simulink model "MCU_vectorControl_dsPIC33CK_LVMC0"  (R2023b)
settings: Solver=FixedStepDiscrete  StartTime=0.0  StopTime=10.0  FixedStep=5e-5  RelTol=1e-3  EnableMultiTasking=on
undefined symbols (not defined in the file or in its folder): A0, A4, ADC, address, also, AN0, AN1, as, B0, B2, below, Bias1, Bias2, bit, bits, BOR, C12, C13, C14, C7, C8, cause, Code, Communicate, control, counter, Custom, D11, D12, D13, D14, D2, D5, D6, D7, D9, dead, default, deviced, diff, disasserted, DiscIntNeverNeededParam, ECIO, ensure, events, faster, HS3, I, I2C, I2C1, I2C2, I2C3, illegalInstruction, Interval, inverter, is, IsSigned1, IsSigned2, kHz, Lowest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
libraries: simulink x55, MCHP_Blockset x25
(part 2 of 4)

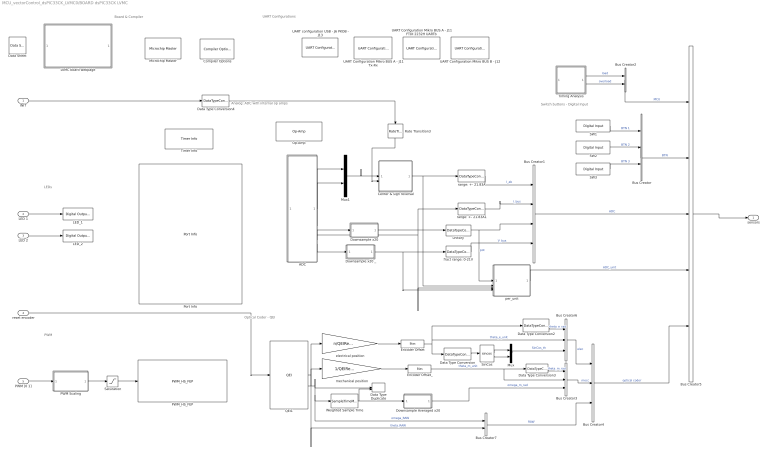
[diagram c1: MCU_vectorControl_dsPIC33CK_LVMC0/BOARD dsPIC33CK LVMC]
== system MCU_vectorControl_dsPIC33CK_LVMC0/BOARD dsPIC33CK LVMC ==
  note: Board & Compiler
  note: Analog: ADC with internal op amps
  note: Optical Coder - QEI
  note: PWM
  note: UART Configurations
  note: LEDs
  note: Switch buttons - Digital Input
  INIT : Inport
  LED 1 : Inport  Port=2
  LED 2 : Inport  Port=3
  reset encoder : Inport  Port=4
  PWM [0 1] : Inport  Port=5  Unit=1
  ADC : Subsystem
  Bus Creator{,3..4,6} (4 alike) : BusCreator  Inputs=3
  Bus Creator1 : BusCreator  Inputs=4
  Bus Creator2 : BusCreator  Inputs=2
  Bus Creator5 : BusCreator  Inputs=5
  Bus Creator7 : BusCreator  Inputs=2
  Center & sign reversal : Subsystem
  Compiler Options : MCHP_Blockset/System Configuration/Compiler Options  Priority=1  LATEST_CMPLR=on  COMP_LIST_TXT=XC16 - v2.10  DFP_LIST_TXT=from compiler  CMSIS_DSP_TXT=Dynamic Options  USE_64BIT_DOUBLE=off  MCHP_MULTITHREAD_COMPILATION=on  UseCustom_LinkerScript=off  MCHP_MASTERLINK=MCU_vectorControl_dsPIC33CK_LVMC0/BOARD dsPIC33CK LVMC/Microchip Master  OPTIMIZATION_LEVEL=2  MPLAB_LINKLIB=relaxed floating-point math  MPLAB_LINKLIB1=default  CodeReplacement_TXT=Microchip Code Replacement Library for dsPIC  OPTIMIZATION_FLTO=on  OPTIMIZATION_REORDER=off  OPTIMIZATION_ASM_REORDER=off  UNROLL_LOOPS=off  PROCEDURAL_ABSTRACTION=off  GC_SECTIONS=None  MCODE=is more than 32768  MCONST=in code memory  MDATA=Can use all available memory  MSCALAR=Use only memory below address 8192 (faster)  MLARGEARRAY=off  MAGGREGATE=on  HEAP_SIZE=0  OMF=elf  DEBUG_INFO=on  MCHP_STACK_USAGE=off  GCC_STACK_USAGE=off  ProduceHexOutput=on  AssemblyListing=off  SaveTemps=off  NO_EDS_WARN=on  PRINT_STATISTICS=off
  Data Sheet : MCHP_Blockset/System Info/Data Sheet  DOC_Type=datasheet  DOC_MCHP_Id=33FJ64MC802  DOC_FileLastCheckTime=[0 0 0 0 0 0]  cpy_MCHP_Id=33CK256MP508  MCHP_MASTERLINK=MCU_vectorControl_dsPIC33CK_LVMC0/BOARD dsPIC33CK LVMC/Microchip Master
  Data Type Duplicate : DataTypeDuplicate
  Data Type Conversion : DataTypeConversion
  Data Type Conversion2 : DataTypeConversion  OutDataTypeStr=fixdt(1,16,(2*pi)/2^16,0)  ConvertRealWorld=Stored Integer (SI)
  Data Type Conversion3 : DataTypeConversion  OutDataTypeStr=fixdt(1,16,(2*pi)/2^16,0)  ConvertRealWorld=Stored Integer (SI)
  Data Type Conversion4 : DataTypeConversion  OutDataTypeStr=boolean
  Downsample Averaged x20 : Subsystem  mask{DownSample=10}
      mask prompts: DownSample "DownSample Factor"
  Downsample x20 : Subsystem  mask{DownSample=20}
      mask prompts: DownSample "DownSample Factor"
  Downsample x20 _ : Subsystem  mask{DownSample=20}
      mask prompts: DownSample "DownSample Factor"
  Encoder Offset : Bias  Bias=mod(1,round((n*QEIOffset)/(2*pi)))
  Encoder Offset_ : Bias  Bias=mod(1,round(QEIOffset/(2*pi)))
  LED_1 : MCHP_Blockset/Digital IO/Digital Output Write  PORT_TXT="E   [ 0 : 15 ]"  PIN=6  INIT_VALUE=-1  PACK=off  OUTPUT_PIN_MODE=Push-Pull (default)  SIMULTANEOUS=off  ORDERING=None  SampleTime=-1  MCHP_PORT={Digital Out}{DOU}1:1:E6;  MCHP_MASTERLINK=MCU_vectorControl_dsPIC33CK_LVMC0/BOARD dsPIC33CK LVMC/Microchip Master
  LED_2 : MCHP_Blockset/Digital IO/Digital Output Write  PORT_TXT="E   [ 0 : 15 ]"  PIN=7  INIT_VALUE=-1  PACK=off  OUTPUT_PIN_MODE=Push-Pull (default)  SIMULTANEOUS=off  ORDERING=None  SampleTime=-1  MCHP_PORT={Digital Out}{DOU}1:1:E7;  MCHP_MASTERLINK=MCU_vectorControl_dsPIC33CK_LVMC0/BOARD dsPIC33CK LVMC/Microchip Master
  LVMC board webpage : Subsystem
  Microchip Master : MCHP_Blockset/System Configuration/Microchip Master  Priority=1  PICREF=33CK256MP508  TIMESTEP_REF=PWM1 Trigger 1 + ADC  BUSYFLAG=Dynamic Options  BUSYFLAG_TXT=None  VDD_range=Dynamic Options  PWRTEN=Not used  BOREN=Disable  BODENV=2.7V  BORV=Not used  FPWRT=128ms  DSBOREN=Enable ZPBOR during Deep Sleep Mode  DSLPBOR=Not used  MCLRE=Enabled  SMCLR=MCLR pin generates a normal system Reset  PMDL1WAY=Allow only one reconfiguration  RSTPRI=Device will obtain reset instruction from Primary flash  TEMP=Not used  SOSCSRC=Not used  SOSCSEL=Not used  IOL1WAY=Allow only one reconfiguration  ALTVREF=Not used  DISUVREG=Not used  DSSWEN=Not used  LPCFG=Not used  RTCBAT=Not used  VBTBOR=Not used  WUTSEL=Not used  POWERSAVE=off  FNOSC=Internal Fast RC (FRC)  FPR=ECIO w/ PLL 16x  FOSFPR=HS3 w/PLL 16x  FOS=Primary Oscillator  FRANGE=High Range  OSCILLATOR_SELECT=Internal Fast RC (FRC)  OSCILLATOR_SELECT_spd=Internal Fast RC (FRC)  QUARTZ=8e6  QUARTZ_spd=8e6  POSCGAIN=2x gain setting  POSCBOOST=Boost the kick start of the oscillator  SOSCGAIN=2x gain setting  SOSCBOOST=Boost the kick start of the oscillator  ACTIV_PLL=on  ACTIV_PLL_spd=on  MIPS_DESIRED=100e6  MIPS_DESIRED_spd=100e6  CPUDIV=Divide by 1  FPLLMUL=Not used  FPLLIDIV=8x Divider  POSCFREQ=Not used  POSCMD=Primary Oscillator Disabled  POSCMOD=Primary Oscillator Disabled  MIPS=100 * 1e6  ACLKCON=Optimized for PWM resolution & ADC conversion speed  ACLKCON_spd=Optimized for PWM resolution & ADC conversion speed  FPLLODIV=32x Divider  PLLKEN=PLL lock signal will be used to disable PLL clock output if lock is lost  FCKSM=Clock switching is enabled;Fail-safe Clock Monitor is disabled  FCKSMEN=Sw Disabled; Mon Disabled  IESO=Start up with FRC; then switch  DSWDTPS=1:2^36  FWDTEN=WDT controlled via SW; use WDTCON.ON bit  FWDTWINSZ=Window size is 25%  FWPSA=1:512  FWPSA0=1:128  FWPSB=1:16  WDT=Disable  WDTPOST=1:32768  WDTPRE=1:128  WDTPS=1:32768  WINDIS=Watchdog Timer operates in Non-Window mode  WWDTEN=Non-Window mode  DSWDTEN=Enable DSWDT during Deep Sleep Mode  DSWDTOSC=Select LPRC as DSWDT Reference clock  FWDT_RCLKSEL=WDT Run Mode uses BFRC:256  FWDT_RWDTPS=1:2147483648  FWDT_SWDTMPS=1:2147483648  FWDT_WDTEN=WDT is controlled by software; use WDTCON.ON bit  FWDT_WDTRSTEN=WDT event generates a reset  FWDT_WDTWIN=WDT Window is 25% of WDT period  FWDT_WINEN=Not used  FPBDIV=Not used  FSOSCEN=Disable Secondary Oscillator  LPRCSEL=Not used  OSCIOFCN=Not used  OSCIOFNC=general purpose digital I/O pin  LVRCFG=Not used  PLL_96MHZ=Not used  PLL96MHZ=Not used  PLLDIV=Not used  WDTCLK=Not used  WDTCMX=Not used  WDTWIN=WDT Window is 25% of WDT period  XTCFG=24-32 MHz crystals  XTBST=Boost the kick-start  APL=Aux Flash Code protect is disabled  APLK=Aux Flash Write Protection or Code Protection is Enabled  AWRP=Auxiliary program memory is not write-protected  BSS=No Protection (other than BWRP)  BWP=Not used  BWRP=Boot Segment may be written  CP=Protection Disabled  EBS=No Boot EEPROM  ESS=No Segment Data EEPROM  GCP=General Segment Code protect is Disabled  GSS=No Protection (other than GWRP)  GSS0=Not used  GSSK=General Segment Write Protection or Code Protection is Enabled  GWRP=General Segment may be written  PWP=Not used  RBS=No Boot RAM  RSS=No Secure RAM  SSS=No Secure Segment  SWRP=Secure segment may be written  WPCFG=Not used  WPDIS=Not used  WPEND=Not used  WPFP=Not used  ICESEL=Communicate on PGEC1/PGED1  ICS=Communicate on PGC3 and PGD3  JTAGEN=Disable  FICD_JTAGEN=Disable  COE=Not used  RES=Not used  DEBUG=Debugger is disabled  BACKBUG=Not used  BKBUG=Not used  ALTI2C=I2C mapped to SDA1/SCL1 pins  ALTI2C1=I2C1 mapped to SDA1/SCL1 pins  ALTI2C2=I2C2 mapped to SDA2/SCL2 pins  ALTI2C3=I2C3 mapped to SDA3/SCL3 pins  FDEVOPT1_ALTI2C1=Not used  FDEVOPT1_ALTI2C2=Not used  FDEVOPT1_SPI2MAPDIS=Not used  FDEVOPT_ALTI2C1=Primary I2C1 pins are used  FDEVOPT_ALTI2C2=Primary I2C2 pins are used  FDEVOPT_ALTI2C3=Primary I2C3 pins are used  FDEVOPT_SPI2PIN=SPI2 pins are selected by peripheral pin selection feature  ALTQIO=QEA1; QEB1; INDX1 are selected as inputs to QEI1  ALTSS1=SS1A is selected as the I/O pin for SPI1  CMPPOL0=Hysteresis is applied to falling edge  CMPPOL1=Hysteresis is applied to falling edge  FCANIO=Not used  FETHIO=Default Ethernet I/O  FMIIEN=MII Enabled  FSRSSEL=Not used  FUSBIDIO=Controlled by the USB Module  FVBUSONIO=Not used  HPOL=PWM module high side output pins have active-high output polarity  HYST0=45 mV Hysteresis  HYST1=45 mV Hysteresis  I2C1SEL=Not used  LPOL=PWM module low side output pins have active-high output polarity  PWMPIN=PWM module pins controlled by PORT register at device Reset  RTCOSC=Not used  UPLLEN=USB PLL Disabled  UPLLIDIV=Not used  ATMOD8=Not used  ALTPMP=Not used  I2C2SEL=Not used  ALTADREF=Not used  ALTCVREF=Not used  PWMLOCK=PWM registers may be written without key sequence  INT_PRIORITY_DMA=0  MCHP_TIMER_RESULT=[ ]  MCHP_PLLRegisters="[1    100  16387     -1     33]"  MCHPVAR=MCHP.fcy.MIPS=1e+08;MCHP.fcy.SYSCLK=1e+08;MCHP.fcy.Fplli=8000000;MCHP.fcy.Fvco=8e+08;MCHP.fcy.Fpllo=4e+08;MCHP.fcy.ADC=1e+08;MCHP.fcy.Comparator=1e+08;MCHP.fcy.I2C=1e+08;MCHP.fcy.SPI=1e+08;MCHP.fcy.UART=2e+08;MCHP.fcy.Timers=1e+08;MCHP.fcy.OC=1e+08;MCHP.fcy.IC=1e+08;MCHP.fcy.Ports=1e+08;MCHP.fcy.QEI=1e+08;MCHP.fcy.APLL=-1;MCHP.PowerSave=0;MCHP.TimeStepFactor=-20000;MCHP.TimeStep_Timer=-1;MCHP.NTIM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  MCHP_CRC=20015258  BTMODE=Device is in Single Boot (legacy) mode  RES1=Not used  PLLSS=Not used  RES2=Not used  ALTCMPI=Not used  BOREN1=Not used  ALTRB6=Not used  RETCFG=Not used  DFMCY=Not used  BSS2=No Boot Segment  BSEN=No Boot Segment  CWRP=Configuration Segment may be written  CSS=No Protection (other than CWRP)  AIVTDIS=Disabled AIVT  BSLIM=Not used  WDTEN=Disable  BTSWP=BOOTSWP instruction is disabled  DBCC=No Cross Connection between DAC outputs  CTXT1=Not Assigned  CTXT2=Not Assigned  SEQNUM=Not used  nSEQNUM=Not used  BOREN0=Enabled  DMTIVT=Not used  DMTCNT=2^31 (2147483648)  DMTEN=Dead Man Timer is Disabled and can be enabled by software  ON=Not used  USERID=Not used  RESERVED1=Not used  PGL1WAY=Allow only one reconfiguration  FPLLRNG=34-68 MHz Input  FPLLICLK=FRC is input to the System PLL  FPLLMULT=PLL Multiply by 128  UPLLFSEL=USB PLL input is 24 MHz  DMTINTV=Window/Interval value is 127/128 counter value  WDTSPGM=WDT stops during Flash programming  FDMTEN=Deadman Timer is disabled  TRCEN=Trace features in the CPU are enabled  BOOTISA=Boot code and Exception code is MIPS32  FECCCON=ECC and Dynamic ECC are disabled (ECCCON bits are writable)  EXTDDRSIZE=Not used  FSLEEP=Flash is powered down when the device is in Sleep mode  DBGPER=Allow CPU access to all permission regions  EJTAGBEN=Normal EJTAG functionality  TSEQ=Not used  CSEQ=Not used  RWDTPS=1:1048576  RCLKSEL=Always use LPRC  SWDTPS=1:1048576  DMTIVTL=Not used  DMTIVTH=Not used  DMTCNTL=Not used  DMTCNTH=Not used  DMTDIS=Dead Man Timer is Disabled and can be enabled by software  SMBEN=SMBus input threshold is enabled  SPI2PIN=SPI2 uses I/O remap (PPS) pins  CTXT3=Not Assigned  CTXT4=Not Assigned  MBXM0=Mailbox register configured for Main data read (Secondary to Main data transfer)  MBXM1=Mailbox register configured for Main data read (Secondary to Main data transfer)  MBXM2=Mailbox register configured for Main data read (Secondary to Main data transfer)  MBXM3=Mailbox register configured for Main data read (Secondary to Main data transfer)  MBXM4=Mailbox register configured for Main data read (Secondary to Main data transfer)  MBXM5=Mailbox register configured for Main data read (Secondary to Main data transfer)  MBXM6=Mailbox register configured for Main data read (Secondary to Main data transfer)  MBXM7=Mailbox register configured for Main data read (Secondary to Main data transfer)  MBXM8=Mailbox register configured for Main data read (Secondary to Main data transfer)  MBXM9=Mailbox register configured for Main data read (Secondary to Main data transfer)  MBXM10=Mailbox register configured for Main data read (Secondary to Main data transfer)  MBXM11=Mailbox register configured for Main data read (Secondary to Main data transfer)  MBXM12=Mailbox register configured for Main data read (Secondary to Main data transfer)  MBXM13=Mailbox register configured for Main data read (Secondary to Main data transfer)  MBXM14=Mailbox register configured for Main data read (Secondary to Main data transfer)  MBXM15=Mailbox register configured for Main data read (Secondary to Main data transfer)  MBXHSA=MSIxMBXD15 assigned to mailbox handshake protocol block A  MBXHSB=MSIxMBXD15 assigned to mailbox handshake protocol block B  MBXHSC=MSIxMBXD15 assigned to mailbox handshake protocol block C  MBXHSD=MSIxMBXD15 assigned to mailbox handshake protocol block D  MBXHSE=MSIxMBXD15 assigned to mailbox handshake protocol block E  MBXHSF=MSIxMBXD15 assigned to mailbox handshake protocol block F  MBXHSG=MSIxMBXD15 assigned to mailbox handshake protocol block G  MBXHSH=MSIxMBXD15 assigned to mailbox handshake protocol block H  HSAEN=Mailbox data flow control handshake protocol block disabled  HSBEN=Mailbox data flow control handshake protocol block disabled  HSCEN=Mailbox data flow control handshake protocol block disabled  HSDEN=Mailbox data flow control handshake protocol block disabled  HSEEN=Mailbox data flow control handshake protocol block disabled  HSFEN=Mailbox data flow control handshake protocol block disabled  HSGEN=Mailbox data flow control handshake protocol block disabled  HSHEN=Mailbox data flow control handshake protocol block disabled  CPRA0=Main core owns pin  CPRA1=Main core owns pin  CPRA2=Main core owns pin  CPRA3=Main core owns pin  CPRA4=Main core owns pin  CPRB0=Main core owns pin  CPRB1=Main core owns pin  CPRB2=Main core owns pin  CPRB3=Main core owns pin  CPRB4=Main core owns pin  CPRB5=Main core owns pin  CPRB6=Main core owns pin  CPRB7=Main core owns pin  CPRB8=Main core owns pin  CPRB9=Main core owns pin  CPRB10=Main core owns pin  CPRB11=Main core owns pin  CPRB12=Main core owns pin  CPRB13=Main core owns pin  CPRB14=Main core owns pin  CPRB15=Main core owns pin  CPRC0=Main core owns pin  CPRC1=Main core owns pin  CPRC2=Main core owns pin  CPRC3=Main core owns pin  CPRC4=Main core owns pin  CPRC5=Main core owns pin  CPRC6=Main core owns pin  CPRC7=Main core owns pin  CPRC8=Main core owns pin  CPRC9=Main core owns pin  CPRC10=Main core owns pin  CPRC11=Main core owns pin  CPRC12=Main core owns pin  CPRC13=Main core owns pin  CPRC14=Main core owns pin  CPRC15=Main core owns pin  CPRD0=Main core owns pin  CPRD1=Main core owns pin  CPRD2=Main core owns pin  CPRD3=Main core owns pin  CPRD4=Main core owns pin  CPRD5=Main core owns pin  CPRD6=Main core owns pin  CPRD7=Main core owns pin  CPRD8=Main core owns pin  CPRD9=Main core owns pin  CPRD10=Main core owns pin  CPRD11=Main core owns pin  CPRD12=Main core owns pin  CPRD13=Main core owns pin  CPRD14=Main core owns pin  CPRD15=Main core owns pin  CPRE0=Main core owns pin  CPRE1=Main core owns pin  CPRE2=Main core owns pin  CPRE3=Main core owns pin  CPRE4=Main core owns pin  CPRE5=Main core owns pin  CPRE6=Main core owns pin  CPRE7=Main core owns pin  CPRE8=Main core owns pin  CPRE9=Main core owns pin  CPRE10=Main core owns pin  CPRE11=Main core owns pin  CPRE12=Main core owns pin  CPRE13=Main core owns pin  CPRE14=Main core owns pin  CPRE15=Main core owns pin  S1FNOSC=Internal Fast RC (FRC) Oscillator with postscaler  S1IESO=Start up with FRC; then switch  S1OSCIOFNC=OSC2 is clock output  S1FCKSM=Both Clock switching and Fail-safe Clock Monitor are disabled  S1PLLKEN=S1PLLKEN_ON  S1RWDTPS=1:1048576  S1RCLKSEL=Always use LPRC  S1WINDIS=Watchdog Timer operates in Non-Window mode  S1WDTWIN=WDT Window is 25% of WDT period  S1SWDTPS=1:1048576  S1FWDTEN=use WDTCON.ON bit  S1ICS=Communicate on PGC3 and PGD3  S1DEBUG=Not used  S1ISOLAT=The Secondary can operate (in debug mode) even if the SLVEN bit in the MSI is zero  S1NOBTSWP=BOOTSWP instruction is disabled  S1ALTI2C1=I2C1 mapped to SDA1/SCL1 pins  S1SPI1PIN=Secondary SPI1 uses I/O remap (PPS) pins  S1SSRE=Secondary generated resets will reset the Secondary Enable Bit in the MSI module  S1MSRE=The Main software oriented RESET events (RESET Op-Code; Watchdog timeout; TRAP reset; illegalInstruction) will also cause the Secondary subsystem to reset  S1CTXT1=Not Assigned  S1CTXT2=Not Assigned  S1CTXT3=Not Assigned  S1CTXT4=Not Assigned  BORLVL=BOR trip point is 2.96 V  BSSO=Normal startup operation after reset; execute instruction at 0x000000  MCA=Flash read accesses are 2 cycle to support maximum processor frequency of operation  MAXTEMP=20 ns flash access  CFGAN14=Device pin is input to AN14  CFGAN15=Device pin is input to AN15  S1IOL1WAY=Allow only one reconfiguration  S1BSSO=Normal startup operation after reset; execute instruction at 0x000000  S1BACKBUG=Not used  BISTDIS=mBIST on reset feature disabled  NOBTSWP=BOOTSWP instruction is disabled  S1BISTDIS=Secondary BIST on reset feature disabled  S1DMTIVTL=Not used  S1DMTIVTH=Not used  S1DMTCNTL=Not used  S1DMTCNTH=Not used  S1DMTDIS=Secondary Dead Man Timer is Disabled and can be enabled by software  BSEQ=Not used  IBSEQ=Not used  SMB3EN=SMBus 3.0 input levels  FUSBIDIO2=USBID pin is controlled by the USB2 module  FVBUSIO2=VBUSON pin is controlled by the USB2 module  FUSBIDIO1=USBID pin is controlled by the USB1 module  FVBUSIO1=VBUSON pin is controlled by the USB1 module  VBATBOREN=Enable ZPBOR during VBAT Mode  FDSEN=Enable DSEN bit in DSCON  BORSEL=BOR trip voltage 2.1v (Non-OPAMP deviced operation)  POSCFGAIN=Gain is G3  POSCAGCDLY=Settling time = 25ms x AGCRNG  POSCAGCRNG=Range 1x  POSCAGC=Automatic Gain Control for Oscillator  FDBGWP=Not used
  Mux : Mux  Inputs=2
  Mux1 : Mux  Inputs=2
  Op-Amp : MCHP_Blockset/Analog IO/Op-Amp  Priority=-2000  OpAmp1=Enabled with positive and negative inputs  OpAmp2=Enabled with positive and negative inputs  OpAmp3=Enabled with positive and negative inputs  S_INPUT=[-1]  S_INPUT_Size=[3]  S_OUTPUT=[]  S_OUTPUT_Size=[]  S_ListCustomDatatype=S.S_ListCustomDatatype={};  MCHP_USER_INTERRUPTS=0  MCHP_PORT={OA1 Output}{OA1out}14:2:A0;{OA1 IN+}{OA1in+}14:2:A2;{OA1 IN-}{OA1in-}14:2:A1;{OA2 Output}{OA2out}14:2:B2;{OA2 IN+}{OA2in+}14:2:B4;{OA2 IN-}{OA2in-}14:2:B3;{OA3 Output}{OA3out}14:2:A4;{OA3 IN+}{OA3in+}14:2:C2;{OA3 IN-}{OA3in-}14:2:C1;  MCHP_MASTERLINK=MCU_vectorControl_dsPIC33CK_LVMC0/BOARD dsPIC33CK LVMC/Microchip Master  MCHP_CRC=1127818
  PWM Scaling : Subsystem
  PWM_HS_FEP : MCHP_Blockset/PWM IO/PWM_HS_FEP  Priority=-2000  PWMx_MODSEL=Center Aligned  PWMx_CLKSEL=no scaling  PWM_ClockResolution_DIVSEL_TXT=auto  PWM_ClockResolution_FSCL_TXT=auto - best resolution  PWM_ClockResolution_NoScaling_TXT="Resol: 0.005(us)  -  MaxPer: 0.000328(s)"  MaxPeriod_s=50e-6  InitPeriode_s=50e-6  InitDutyCycleP_s=25e-6  InitDutyCycleS_s=10e-6  InitPhase_s=-1  evalin_ws=PWM1max=MCHP_Fun.Hex2num('40B3880000000000');PWM2max=MCHP_Fun.Hex2num('40B3880000000000');PWM4max=MCHP_Fun.Hex2num('40B3880000000000');  SampleTime=-1  S_INPUT=[-1]  S_INPUT_Size=[3]  S_OUTPUT=[]  S_OUTPUT_Size=[]  S_ListCustomDatatype=S.S_ListCustomDatatype={};  MCHP_USER_INTERRUPTS=0  MCHP_PORT={PWMH1 }{PWMH1}32:4:B14;{PWMH2 }{PWMH2}32:4:B12;{PWMH4 }{PWMH4}32:4:D1;{PWML1}{PWML1}32:4:B15;{PWML2}{PWML2}32:4:B13;{PWML4}{PWML4}32:4:D0;  MCHP_MASTERLINK=MCU_vectorControl_dsPIC33CK_LVMC0/BOARD dsPIC33CK LVMC/Microchip Master  MCHP_CRC=5297627  PWMx_PMOD=Complementary  PWM1_HL=PWMxH & PWMxL output enabled  PWM1_swap=off  PWM1H_pol=off  PWM1L_pol=off  PWM2_HL=PWMxH & PWMxL output enabled  PWM2_swap=off  PWM2H_pol=off  PWM2L_pol=off  PWM3_HL=not used  PWM3_swap=off  PWM3H_pol=off  PWM3L_pol=off  PWM4_HL=PWMxH & PWMxL output enabled  PWM4_swap=off  PWM4H_pol=off  PWM4L_pol=off  PWM5_HL=not used  PWM5_swap=off  PWM5H_pol=off  PWM5L_pol=off  PWM6_HL=not used  PWM6_swap=off  PWM6H_pol=off  PWM6L_pol=off  PWM7_HL=not used  PWM7_swap=off  PWM7H_pol=off  PWM7L_pol=off  PWM8_HL=not used  PWM8_swap=off  PWM8H_pol=off  PWM8L_pol=off  PWM9_HL=not used  PWM9_swap=off  PWM9H_pol=off  PWM9L_pol=off  PWM10_HL=not used  PWM10_swap=off  PWM10H_pol=off  PWM10L_pol=off  PWM11_HL=not used  PWM11_swap=off  PWM11H_pol=off  PWM11L_pol=off  PWM12_HL=not used  PWM12_swap=off  PWM12H_pol=off  PWM12L_pol=off  PWM1_ShowTrig=on  PWM1_Init_PGxTRIGABC_s=[0 -1 -1 ]  PWM1_ADTRxEN1=ADC Trigger 1  PWM1_ADTRxEN2=none  PWM1_ADTRxEN3=none  PWM2_ShowTrig=off  PWM2_Init_PGxTRIGABC_s=[-1 -1 -1]  PWM2_ADTRxEN1=none  PWM2_ADTRxEN2=none  PWM2_ADTRxEN3=none  PWM3_ShowTrig=off  PWM3_Init_PGxTRIGABC_s=[-1 -1 -1]  PWM3_ADTRxEN1=none  PWM3_ADTRxEN2=none  PWM3_ADTRxEN3=none  PWM4_ShowTrig=off  PWM4_Init_PGxTRIGABC_s=[-1 -1 -1]  PWM4_ADTRxEN1=none  PWM4_ADTRxEN2=none  PWM4_ADTRxEN3=none  PWM5_ShowTrig=off  PWM5_Init_PGxTRIGABC_s=[-1 -1 -1]  PWM5_ADTRxEN1=none  PWM5_ADTRxEN2=none  PWM5_ADTRxEN3=none  PWM6_ShowTrig=off  PWM6_Init_PGxTRIGABC_s=[-1 -1 -1]  PWM6_ADTRxEN1=none  PWM6_ADTRxEN2=none  PWM6_ADTRxEN3=none  PWM7_ShowTrig=off  PWM7_Init_PGxTRIGABC_s=[-1 -1 -1]  PWM7_ADTRxEN1=none  PWM7_ADTRxEN2=none  PWM7_ADTRxEN3=none  PWM8_ShowTrig=off  PWM8_Init_PGxTRIGABC_s=[-1 -1 -1]  PWM8_ADTRxEN1=none  PWM8_ADTRxEN2=none  PWM8_ADTRxEN3=none  BlockInput_VectorScalar=Vectors (grouped by function)  BlockInput_Period=Not a block input  BlockInput_DutyCycle=a Uint raw input (PWMxmax variable represent max period)  BlockInput_PhaseShift=Not a block input  BlockInput_SEVTCMP=Not a block input  BlockInput_TRIGx=Not a block input  BlockInput_DeadTime=Not a block input  BlockOutput_FaultDisabled=off  BlockOutput_Fault=on  DTC=Positive dead time (ensure period of time with PWM_H and PWM_L disasserted)  FLTSRC1_DTCMP_TXT=<empty>  FLTSRC2_DTCMP_TXT=<empty>  FLTSRC3_DTCMP_TXT=<empty>  FLTSRC4_DTCMP_TXT=<empty>  FLTSRC5_DTCMP_TXT=<empty>  FLTSRC6_DTCMP_TXT=<empty>  FLTSRC7_DTCMP_TXT=<empty>  FLTSRC8_DTCMP_TXT=<empty>  FLTSRC9_DTCMP_TXT=<empty>  FLTSRC10_DTCMP_TXT=<empty>  FLTSRC11_DTCMP_TXT=<empty>  FLTSRC12_DTCMP_TXT=<empty>  DeadTime_s=1e-6  DeadTimeAlt_s=1e-6  DeadTimeComp_s=0  FLTMODx=Disabled  FLTSRCx_TXT=<empty>  FLTDATx=PWM H/L -> 11  CLMODx=Disabled  CLSRCx_TXT=<empty>  CLDATx=PWM H/L -> 00  FLTLEBENx=off  CLLEBENx=off  LeadEdgeBlkPer_s=5e-7  PHRx=off  PHFx=off  PLRx=off  PLFx=off
  Port Info : MCHP_Blockset/System Info/Port Info  MCHP_MASTERLINK=MCU_vectorControl_dsPIC33CK_LVMC0/BOARD dsPIC33CK LVMC/Microchip Master
  QEI1 : MCHP_Blockset/QEI/QEI  QEI_REF=1  QEI_MODE=Quadrature Encoder  QEI_x2mode=off  QEI_PulseCountDir=Down  PIN_QEA_TXT=C12 / P60 / Pin[5]  PIN_QEB_TXT=C13 / P61 / Pin[6]  SWPAB=on  QEAPOL=off  QEBPOL=off  SampleTime=50e-6  PIN_CCMP_TXT=A4 / P20 / Pin[33]  MCHP_PORT={QEI1 A}{QEIA1}5:0:P60;{QEI1 B}{QEIB1}5:0:P61;  MCHP_MASTERLINK=MCU_vectorControl_dsPIC33CK_LVMC0/BOARD dsPIC33CK LVMC/Microchip Master  INDXxCNT_Output=is not an output  POSxCNT_Output=is a 16 bits signed block output  RESET_Input=on  PIMOD_mode=position is cyclique between user defined boundaries  PIMOD_modeB=Never reset position  PIMOD_reset=on next INDEX event  PIN_INDEX_TXT=C14 / P62 / Pin[7]  IMV=QEA = 0 and QEB = 0  IMV_x2=QEA = 1  PIN_HOME_TXT=B0 / P32 / Pin[34]  QEIxLEC_GEC=[0 (QEIResolution-1)]  QEIxIC=0  PCIIRQ=off  IDXPOL=on  HOMPOL=on  VELxCNT_Output=is a 16 bits signed block output  INTxHLD_Output=is not an output  MaxPeriod=1e-3  FILTREN=on  QFDIV_popup_TXT=8333.33 kHz  FILTER_CutOffFreq=100e3  QEI_IntPri=5
  Rate Transition3 : RateTransition  Deterministic=off
  SW1 : MCHP_Blockset/Digital IO/Digital Input  PORT_TXT="E   [ 0 : 15 ]"  PIN=11  INPUT_PIN_MODE=Hi-impedance (default)  PACK=off  SIMULTANEOUS=off  ORDERING=None  SampleTime=-1  MCHP_PORT={Digital In}{DIN}2:0:E11;  MCHP_MASTERLINK=MCU_vectorControl_dsPIC33CK_LVMC0/BOARD dsPIC33CK LVMC/Microchip Master
  SW2 : MCHP_Blockset/Digital IO/Digital Input  PORT_TXT="E   [ 0 : 15 ]"  PIN=12  INPUT_PIN_MODE=Hi-impedance (default)  PACK=off  SIMULTANEOUS=off  ORDERING=None  SampleTime=-1  MCHP_PORT={Digital In}{DIN}2:0:E12;  MCHP_MASTERLINK=MCU_vectorControl_dsPIC33CK_LVMC0/BOARD dsPIC33CK LVMC/Microchip Master
  SW3 : MCHP_Blockset/Digital IO/Digital Input  PORT_TXT="E   [ 0 : 15 ]"  PIN=13  INPUT_PIN_MODE=Hi-impedance (default)  PACK=off  SIMULTANEOUS=off  ORDERING=None  SampleTime=-1  MCHP_PORT={Digital In}{DIN}2:0:E13;  MCHP_MASTERLINK=MCU_vectorControl_dsPIC33CK_LVMC0/BOARD dsPIC33CK LVMC/Microchip Master
  Saturation : Saturate  UpperLimit=PWM1max*0.97  LowerLimit=PWM1max*0.03  LinearizeAsGain=off  OutDataTypeStr=uint16
  SinCos : Trigonometry  Operator=sincos  ApproximationMethod=Lookup  AngleUnit=revolution  TableDataTypeStr=fixdt(1,16,14)
  Timer Info : MCHP_Blockset/System Info/Timer Info  MCHP_MASTERLINK=MCU_vectorControl_dsPIC33CK_LVMC0/BOARD dsPIC33CK LVMC/Microchip Master
  Timing Analysis : Subsystem
  UART Configuration Mikro BUS A - J11 FTDI 2232H UARTb : MCHP_Blockset/BUS UART/UART Configuration  UART_REF=3  BAUD_Choice_TXT="3000000         [-0.50%]"  BAUD_Choice_IR_TXT=[]  BAUD_Custom=9000000  INT_PRIORITY=0  ALT_IO=on  PIN_RX_TXT=D12 / P76 / Pin[27]  PIN_RX_INPUT_MODE=Hi-impedance (default)  PIN_TX_TXT=D11 / P75 / Pin[36]  PIN_TX_OUTPUT_MODE=Push-Pull (default)  MCHP_PORT="{UART3  Rx}{U3RX}3:0:P76;{UART3  Tx}{U3TX}3:0:P75;"  MCHP_MASTERLINK=MCU_vectorControl_dsPIC33CK_LVMC0/BOARD dsPIC33CK LVMC/Microchip Master  MCHP_COM_ExtPil=off  TX_IMPLEMENTATION=Circular Buffer  TX_IMPLEMENTATION_default=Circular Buffer  TX_INT_PRIORITY=5  TX_INT_WHEN=has one empty space  TX_INT_WHEN_default=is empty & last char is sent  TX_CIRCULAR_SIZE=1024  TX_DMA_CHANNEL=1  TX_DMA_SIZE=16  TX_TASK_PROTECTION=Delay tasks (default)  TX_INTERRUPT_PROTECTION=Do not send on conflict (default)  TX_INTERRUPT_PROTECTION_default=Do not send on conflict (default)  RX_IMPLEMENTATION=Circular Buffer  RX_IMPLEMENTATION_default=Circular Buffer  RX_INT_PRIORITY=7  RX_INT_WHEN=receive 1 character  RX_CIRCULAR_SIZE=64  RX_DMA_CHANNEL=0  RX_DMA_SIZE=0  DuplexMode=Full duplex (default)  PIN_RX_Inv=off  PIN_TX_Inv=off  PIN_RXTX_Inv=off  ParityBit=No parity (default)  StopBit=1 stop bit (default)  IRDA=off  IdleTime_choice_TXT=None  IdleTime_custom=2/50  FlowControl=None  PIN_CTS_TXT=B0 / P32 / Pin[34]  PIN_CTS_INPUT_MODE=Hi-impedance (default)  PIN_RTS_TXT=B0 / P32 / Pin[34]  PIN_RTS_OUTPUT_MODE=Push-Pull (default)  PIN_DSR_TXT=B0 / P32 / Pin[34]  PIN_DSR_INPUT_MODE=Hi-impedance (default)  PIN_DTR_TXT=B0 / P32 / Pin[34]  PIN_DTR_OUTPUT_MODE=Push-Pull (default)  InitSequence_chkbox=off  BAUD_Choice_InitSeq_TXT="110         [+73.40%]"  BAUD_Choice_IR_InitSeq_TXT=0  BAUD_Custom_InitSeq=0  InitSequence="uint8(['use VT100 terminal ! ' 13 10 27 'c'  27 '[2J' ] )"
  UART Configuration Mikro BUS A - J11 Tx-Rx : MCHP_Blockset/BUS UART/UART Configuration  UART_REF=2  BAUD_Choice_TXT="921600         [+0.01%]"  BAUD_Choice_IR_TXT=[]  BAUD_Custom=5520000  INT_PRIORITY=0  ALT_IO=on  PIN_RX_TXT=D7 / P71 / Pin[52]  PIN_RX_INPUT_MODE=Hi-impedance (default)  PIN_TX_TXT=C7 / P55 / Pin[40]  PIN_TX_OUTPUT_MODE=Push-Pull (default)  MCHP_PORT="{UART2  Rx}{U2RX}3:0:P71;{UART2  Tx}{U2TX}3:0:P55;"  MCHP_MASTERLINK=MCU_vectorControl_dsPIC33CK_LVMC0/BOARD dsPIC33CK LVMC/Microchip Master  MCHP_COM_ExtPil=off  TX_IMPLEMENTATION=DMA Circular Buffer  TX_IMPLEMENTATION_default=Circular Buffer  TX_INT_PRIORITY=5  TX_INT_WHEN=is empty & last char is sent  TX_INT_WHEN_default=is empty & last char is sent  TX_CIRCULAR_SIZE=1024  TX_DMA_CHANNEL=2  TX_DMA_SIZE=16  TX_TASK_PROTECTION=Delay tasks (default)  TX_INTERRUPT_PROTECTION=Do not send on conflict (default)  TX_INTERRUPT_PROTECTION_default=Do not send on conflict (default)  RX_IMPLEMENTATION=Circular Buffer  RX_IMPLEMENTATION_default=Circular Buffer  RX_INT_PRIORITY=7  RX_INT_WHEN=receive 1 character  RX_CIRCULAR_SIZE=64  RX_DMA_CHANNEL=0  RX_DMA_SIZE=0  DuplexMode=Full duplex (default)  PIN_RX_Inv=off  PIN_TX_Inv=off  PIN_RXTX_Inv=off  ParityBit=No parity (default)  StopBit=1 stop bit (default)  IRDA=off  IdleTime_choice_TXT=None  IdleTime_custom=2/50  FlowControl=None  PIN_CTS_TXT=B0 / P32 / Pin[34]  PIN_CTS_INPUT_MODE=Hi-impedance (default)  PIN_RTS_TXT=B0 / P32 / Pin[34]  PIN_RTS_OUTPUT_MODE=Push-Pull (default)  PIN_DSR_TXT=B0 / P32 / Pin[34]  PIN_DSR_INPUT_MODE=Hi-impedance (default)  PIN_DTR_TXT=B0 / P32 / Pin[34]  PIN_DTR_OUTPUT_MODE=Push-Pull (default)  InitSequence_chkbox=off  BAUD_Choice_InitSeq_TXT="110         [+73.40%]"  BAUD_Choice_IR_InitSeq_TXT=0  BAUD_Custom_InitSeq=0  InitSequence="uint8(['use VT100 terminal ! ' 13 10 27 'c'  27 '[2J' ] )"
  UART Configuration Mikro BUS B - J12 : MCHP_Blockset/BUS UART/UART Configuration  Commented=on  UART_REF=3  BAUD_Choice_TXT="8000000         [+0.00%]"  BAUD_Choice_IR_TXT=[]  BAUD_Custom=9000000  INT_PRIORITY=0  ALT_IO=on  PIN_RX_TXT=D5 / P69 / Pin[54]  PIN_RX_INPUT_MODE=Hi-impedance (default)  PIN_TX_TXT=D6 / P70 / Pin[53]  PIN_TX_OUTPUT_MODE=Push-Pull (default)  MCHP_PORT="{UART3  Tx}{U3TX}3:0:P70;"  MCHP_MASTERLINK=MCU_vectorControl_dsPIC33CK_LVMC0/BOARD dsPIC33CK LVMC/Microchip Master  MCHP_COM_ExtPil=off  TX_IMPLEMENTATION=Circular Buffer  TX_IMPLEMENTATION_default=Circular Buffer  TX_INT_PRIORITY=4  TX_INT_WHEN=has one empty space  TX_INT_WHEN_default=is empty & last char is sent  TX_CIRCULAR_SIZE=256  TX_DMA_CHANNEL=2  TX_DMA_SIZE=16  TX_TASK_PROTECTION=Delay tasks (default)  TX_INTERRUPT_PROTECTION=Do not send on conflict (default)  TX_INTERRUPT_PROTECTION_default=Do not send on conflict (default)  RX_IMPLEMENTATION=Do not implement Rx  RX_IMPLEMENTATION_default=Circular Buffer  RX_INT_PRIORITY=7  RX_INT_WHEN=receive 1 character  RX_CIRCULAR_SIZE=64  RX_DMA_CHANNEL=0  RX_DMA_SIZE=0  DuplexMode=Full duplex (default)  PIN_RX_Inv=off  PIN_TX_Inv=off  PIN_RXTX_Inv=off  ParityBit=No parity (default)  StopBit=1 stop bit (default)  IRDA=off  IdleTime_choice_TXT=0  IdleTime_custom=2/50  FlowControl=None  PIN_CTS_TXT=B0 / P32 / Pin[34]  PIN_CTS_INPUT_MODE=Hi-impedance (default)  PIN_RTS_TXT=B0 / P32 / Pin[34]  PIN_RTS_OUTPUT_MODE=Push-Pull (default)  PIN_DSR_TXT=Dynamic Options  PIN_DSR_INPUT_MODE=Hi-impedance (default)  PIN_DTR_TXT=Dynamic Options  PIN_DTR_OUTPUT_MODE=Push-Pull (default)  InitSequence_chkbox=off  BAUD_Choice_InitSeq_TXT="110         [+73.40%]"  BAUD_Choice_IR_InitSeq_TXT=0  BAUD_Custom_InitSeq=0  InitSequence="uint8(['use VT100 terminal ! ' 13 10 27 'c'  27 '[2J' ] )"
  UART configuration USB - J6 PKOB - J13 : MCHP_Blockset/BUS UART/UART Configuration  UART_REF=1  BAUD_Choice_TXT="460800         [+0.01%]"  BAUD_Choice_IR_TXT=[]  BAUD_Custom=115200  INT_PRIORITY=0  ALT_IO=on  PIN_RX_TXT=D14 / P78 / Pin[13]  PIN_RX_INPUT_MODE=Hi-impedance (default)  PIN_TX_TXT=D13 / P77 / Pin[14]  PIN_TX_OUTPUT_MODE=Push-Pull (default)  MCHP_PORT="{UART1  Rx}{U1RX}3:0:P78;{UART1  Tx}{U1TX}3:0:P77;"  MCHP_MASTERLINK=MCU_vectorControl_dsPIC33CK_LVMC0/BOARD dsPIC33CK LVMC/Microchip Master  MCHP_COM_ExtPil=off  TX_IMPLEMENTATION=DMA Circular Buffer  TX_IMPLEMENTATION_default=Circular Buffer  TX_INT_PRIORITY=5  TX_INT_WHEN=is empty  TX_INT_WHEN_default=is empty & last char is sent  TX_CIRCULAR_SIZE=256  TX_DMA_CHANNEL="0   (Lowest Priority)"  TX_DMA_SIZE=512  TX_TASK_PROTECTION=Delay tasks (default)  TX_INTERRUPT_PROTECTION=Do not send on conflict (default)  TX_INTERRUPT_PROTECTION_default=Do not send on conflict (default)  RX_IMPLEMENTATION=Circular Buffer  RX_IMPLEMENTATION_default=Circular Buffer  RX_INT_PRIORITY=7  RX_INT_WHEN=receive 1 character  RX_CIRCULAR_SIZE=64  RX_DMA_CHANNEL=0  RX_DMA_SIZE=0  DuplexMode=Full duplex (default)  PIN_RX_Inv=off  PIN_TX_Inv=off  PIN_RXTX_Inv=off  ParityBit=No parity (default)  StopBit=1 stop bit (default)  IRDA=off  IdleTime_choice_TXT=None  IdleTime_custom=2/50  FlowControl=None  PIN_CTS_TXT=B0 / P32 / Pin[34]  PIN_CTS_INPUT_MODE=Hi-impedance (default)  PIN_RTS_TXT=B0 / P32 / Pin[34]  PIN_RTS_OUTPUT_MODE=Push-Pull (default)  PIN_DSR_TXT=B0 / P32 / Pin[34]  PIN_DSR_INPUT_MODE=Hi-impedance (default)  PIN_DTR_TXT=B0 / P32 / Pin[34]  PIN_DTR_OUTPUT_MODE=Push-Pull (default)  InitSequence_chkbox=off  BAUD_Choice_InitSeq_TXT="115200         [+0.01%]"  BAUD_Choice_IR_InitSeq_TXT=0  BAUD_Custom_InitSeq=0  InitSequence="uint8(['use VT100 terminal ! ' 13 10 27 'c'  27 '[2J' ] )"
  Weighted Sample Time : SampleTimeMath  TsampMathOp=/  weightValue=QEIResolution / (2*pi)  OutDataTypeStr=Inherit: Inherit via back propagation
  electrical position : Gain  Gain=n/QEIResolution  OutDataTypeStr=fixdt(0,16,16)
  fract range: 0-21V : DataTypeConversion  OutDataTypeStr=fixdt(0,16,3.3/65536*21,0)  ConvertRealWorld=Stored Integer (SI)
  mechanical position : Gain  Gain=1/QEIResolution  OutDataTypeStr=fixdt(0,16,16)
  per_unit : Subsystem
  range: +- 21.83A : DataTypeConversion  OutDataTypeStr=fixdt(1,16,21.83/32768,0)  ConvertRealWorld=Stored Integer (SI)
  range: +- 21.83A1 : DataTypeConversion  OutDataTypeStr=fixdt(1,16,21.83/32768,0)  ConvertRealWorld=Stored Integer (SI)
  unitary : DataTypeConversion  OutDataTypeStr=fixdt(0,16,16)  ConvertRealWorld=Stored Integer (SI)
  sensors : Outport
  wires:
  ADC/4(pot) -> Downsample x20/1(In1)
  SW3/1 -> Bus Creator/3  "BTN 3"
  LED 2/1 -> LED_2/1
  SW2/1 -> Bus Creator/2  "BTN 2"
  QEI1/1 -> Bus Creator7/2, mechanical position/1, electrical position/1  "theta_RAW"
  Mux/1 -> Bus Creator6/3  "SinCos_th"
  mechanical position/1 -> Encoder Offset_/1
  ADC/5(V_BUS) -> Downsample x20 _/1(In1)
  Downsample x20/1(Out1) -> unitary/1
  SinCos/1 -> Mux/1
  Saturation/1 -> PWM_HS_FEP/1
  Bus Creator2/1 -> Bus Creator5/1  "MCU"
  ADC/1(Ia) -> Mux1/1
  Bus Creator4/1 -> Bus Creator5/5  "optical coder"
  Bus Creator/1 -> Bus Creator5/2  "BTN"
  SinCos/2 -> Mux/2
  Downsample Averaged x20/1(Out1) -> Bus Creator3/3  "omega_m_rad"
  Data Type Conversion/1 -> SinCos/1
  SW1/1 -> Bus Creator/1  "BTN 1"
  PWM Scaling/1(PWM) -> Saturation/1
  electrical position/1 -> Encoder Offset/1
  Weighted Sample Time/1 -> Data Type Duplicate/2, Downsample Averaged x20/1(In1)
  Timing Analysis/2(CPU Overload) -> Bus Creator2/2  "overload"
  Timing Analysis/1(CPU Load) -> Bus Creator2/1  "load"
  QEI1/2 -> Data Type Duplicate/1, Bus Creator7/1, Weighted Sample Time/1  "omega_RAW"
  range: +- 21.83A/1 -> Bus Creator1/1  "I_ab"
  fract range: 0-21V/1 -> Bus Creator1/4  "V_bus"
  Bus Creator1/1 -> Bus Creator5/3  "ADC"
  INIT/1 -> Data Type Conversion4/1
  ADC/3(IBus) -> range: +- 21.83A1/1, per_unit/3(I_bus)
  ADC/2(Ib) -> Mux1/2
  Bus Creator5/1 -> sensors/1
  PWM [0 1]/1 -> PWM Scaling/1(vabc [0 1])
  Bus Creator3/1 -> Bus Creator4/2  "mecc"
  Bus Creator6/1 -> Bus Creator4/1  "elec"
  LED 1/1 -> LED_1/1
  reset encoder/1 -> QEI1/1
  per_unit/1(ADC_unit) -> Bus Creator5/4  "ADC_unit"
  Data Type Conversion2/1 -> Bus Creator6/1  "theta_e_rad"
  Bus Creator7/1 -> Bus Creator4/3  "RAW"
  range: +- 21.83A1/1 -> Bus Creator1/2  "I_bus"
  unitary/1 -> per_unit/1(pot), Bus Creator1/3  "pot"
  Downsample x20 _/1(Out1) -> per_unit/4(V_bus), fract range: 0-21V/1
  Center & sign reversal/1(Iab) -> range: +- 21.83A/1, per_unit/2(I_ab)
  Rate Transition3/1 -> Center & sign reversal/2(Bias Update)
  Mux1/1 -> Center & sign reversal/1(I_ab)
  Data Type Conversion3/1 -> Bus Creator3/1  "theta_m_rad"
  Encoder Offset/1 -> Bus Creator6/2, Data Type Conversion2/1, Data Type Conversion/1  "theta_e_unit"
  Encoder Offset_/1 -> Bus Creator3/2, Data Type Conversion3/1  "theta_m_unit"
  Data Type Conversion4/1 -> Rate Transition3/1

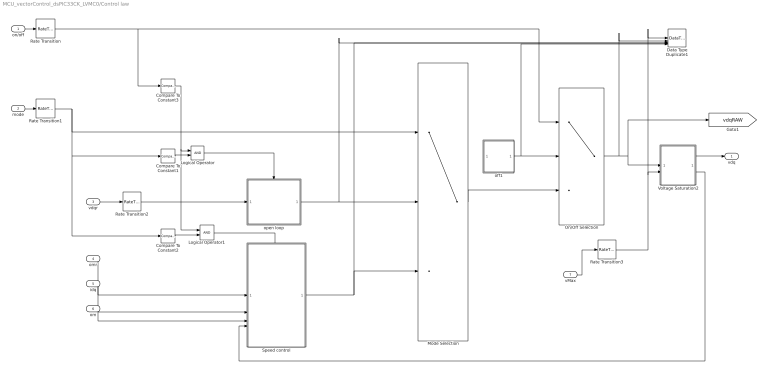
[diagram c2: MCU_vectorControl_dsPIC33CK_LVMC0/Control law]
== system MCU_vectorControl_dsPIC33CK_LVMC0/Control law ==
  on/off : Inport
  mode : Inport  Port=2
  vdqr : Inport  Port=3
  omr : Inport  Port=4
  idq : Inport  Port=5
  om : Inport  Port=6
  vMax : Inport  Port=7
  Compare To Constant1 : simulink/Logic and Bit Operations/Compare To Constant  relop===  const=0  OutDataTypeStr=boolean
  Compare To Constant2 : simulink/Logic and Bit Operations/Compare To Constant  relop===  const=1  OutDataTypeStr=boolean
  Compare To Constant3 : simulink/Logic and Bit Operations/Compare To Constant  relop===  const=1  OutDataTypeStr=boolean
  Data Type Duplicate1 : DataTypeDuplicate  NumInputPorts=5
  Logical Operator : Logic  AllPortsSameDT=off  OutDataTypeStr=boolean
  Logical Operator1 : Logic  AllPortsSameDT=off  OutDataTypeStr=boolean
  Mode Selection : MultiPortSwitch  DataPortOrder=Zero-based contiguous  Inputs=2  DiagnosticForDefault=None  zeroidx=on
  On/Off Selection : MultiPortSwitch  DataPortOrder=Zero-based contiguous  Inputs=2  DiagnosticForDefault=None  zeroidx=on
  Rate Transition{,1..3} (4 alike) : RateTransition
  Speed control : Subsystem
  Voltage Saturation2 : Subsystem
  off1 : Subsystem
  open loop : Subsystem
  vdq : Outport  VectorParamsAs1DForOutWhenUnconnected=off
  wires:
  omr/1 -> Speed control/1(omr)
  Rate Transition2/1 -> open loop/1(vdqr)
  Rate Transition1/1 -> Compare To Constant1/1, Compare To Constant2/1, Mode Selection/1
  Rate Transition/1 -> On/Off Selection/1, Compare To Constant3/1
  Voltage Saturation2/1(vdqsat) -> vdq/1
  mode/1 -> Rate Transition1/1
  Compare To Constant2/1 -> Logical Operator1/2
  Logical Operator/1 -> open loop/Enable
  vMax/1 -> Rate Transition3/1
  Mode Selection/1 -> On/Off Selection/3
  off1/1(vdq) -> Data Type Duplicate1/5, On/Off Selection/2
  open loop/1(vdq) -> Data Type Duplicate1/3, Mode Selection/2
  on/off/1 -> Rate Transition/1
  vdqr/1 -> Rate Transition2/1
  Compare To Constant1/1 -> Logical Operator/2
  Compare To Constant3/1 -> Logical Operator1/1, Logical Operator/1
  Logical Operator1/1 -> Speed control/5(enable)
  om/1 -> Speed control/3(om)
  idq/1 -> Speed control/2(idq)
  Voltage Saturation2/2(saturation) -> Speed control/4(saturation)
  Speed control/1(vdq) -> Data Type Duplicate1/4, Mode Selection/3
  Rate Transition3/1 -> Data Type Duplicate1/1, Voltage Saturation2/2(vMax)
  On/Off Selection/1 -> Data Type Duplicate1/2, [vdqRAW], Voltage Saturation2/1(vdq)

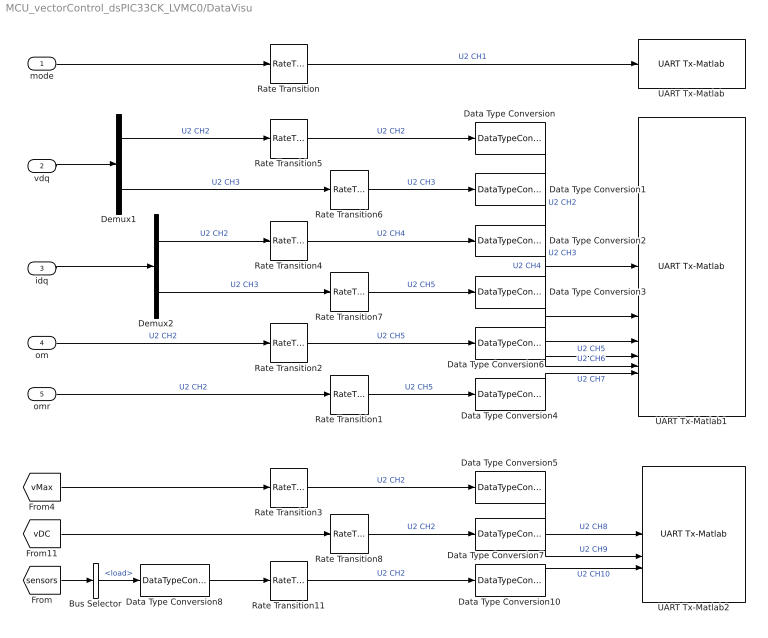
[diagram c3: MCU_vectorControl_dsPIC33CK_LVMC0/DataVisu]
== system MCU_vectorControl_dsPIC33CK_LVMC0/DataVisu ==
  mode : Inport
  vdq : Inport  Port=2
  idq : Inport  Port=3
  om : Inport  Port=4
  omr : Inport  Port=5
  Bus Selector : BusSelector  OutputSignals=MCU.load
  Data Type Conversion{,1..7,10} (9 alike) : DataTypeConversion  OutDataTypeStr=int16  ConvertRealWorld=Stored Integer (SI)
  Data Type Conversion8 : DataTypeConversion  OutDataTypeStr=fixdt(1,16,8)
  Demux1 : Demux  Outputs=2
  Demux2 : Demux  Outputs=2
  Rate Transition{,1..8,11} (10 alike) : RateTransition
  UART Tx-Matlab : MCHP_Blockset/BUS UART/UART Tx-Matlab  UART_REF=2  CHANNELS=[1]  AllOrNothing=off  SampleTime=0.0005  MCHP_MASTERLINK=MCU_vectorControl_dsPIC33CK_LVMC0/BOARD dsPIC33CK LVMC/Microchip Master  MCHP_COMPILED_INFO="CompiledSampleTime= [0.00050000000000000001041   0 ];CompiledInportDataTypes=[  5 ];CompiledInportDataWidth=[1];"
  UART Tx-Matlab1 : MCHP_Blockset/BUS UART/UART Tx-Matlab  UART_REF=2  CHANNELS=[2:7]  AllOrNothing=off  SampleTime=0.0005  MCHP_MASTERLINK=MCU_vectorControl_dsPIC33CK_LVMC0/BOARD dsPIC33CK LVMC/Microchip Master  MCHP_COMPILED_INFO="CompiledSampleTime= [0.00050000000000000001041   0 ];CompiledInportDataTypes=[  4   4   4   4   4   4 ];CompiledInportDataWidth=[1  1  1  1  1  1];"
  UART Tx-Matlab2 : MCHP_Blockset/BUS UART/UART Tx-Matlab  UART_REF=2  CHANNELS=[8:10]  AllOrNothing=off  SampleTime=0.0005  MCHP_MASTERLINK=MCU_vectorControl_dsPIC33CK_LVMC0/BOARD dsPIC33CK LVMC/Microchip Master  MCHP_COMPILED_INFO="CompiledSampleTime= [0.00050000000000000001041   0 ];CompiledInportDataTypes=[  4   4   4 ];CompiledInportDataWidth=[1  1  1];"
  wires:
  Data Type Conversion8/1 -> Rate Transition11/1
  [sensors] -> Bus Selector/1
  Rate Transition11/1 -> Data Type Conversion10/1  "U2 CH2"
  Data Type Conversion10/1 -> UART Tx-Matlab2/3  "U2 CH10"
  Bus Selector/1 -> Data Type Conversion8/1  "<load>"
  Rate Transition8/1 -> Data Type Conversion7/1  "U2 CH2"
  Rate Transition3/1 -> Data Type Conversion5/1  "U2 CH2"
  Data Type Conversion7/1 -> UART Tx-Matlab2/2  "U2 CH9"
  Data Type Conversion5/1 -> UART Tx-Matlab2/1  "U2 CH8"
  [vMax] -> Rate Transition3/1
  [vDC] -> Rate Transition8/1
  Rate Transition1/1 -> Data Type Conversion4/1  "U2 CH5"
  Data Type Conversion4/1 -> UART Tx-Matlab1/6  "U2 CH7"
  omr/1 -> Rate Transition1/1  "U2 CH2"
  mode/1 -> Rate Transition/1
  Rate Transition/1 -> UART Tx-Matlab/1  "U2 CH1"
  om/1 -> Rate Transition2/1  "U2 CH2"
  Data Type Conversion6/1 -> UART Tx-Matlab1/5  "U2 CH6"
  Rate Transition2/1 -> Data Type Conversion6/1  "U2 CH5"
  Data Type Conversion3/1 -> UART Tx-Matlab1/4  "U2 CH5"
  Data Type Conversion2/1 -> UART Tx-Matlab1/3  "U2 CH4"
  Data Type Conversion1/1 -> UART Tx-Matlab1/2  "U2 CH3"
  Data Type Conversion/1 -> UART Tx-Matlab1/1  "U2 CH2"
  Rate Transition7/1 -> Data Type Conversion3/1  "U2 CH5"
  Demux1/1 -> Rate Transition5/1  "U2 CH2"
  Rate Transition4/1 -> Data Type Conversion2/1  "U2 CH4"
  Rate Transition6/1 -> Data Type Conversion1/1  "U2 CH3"
  Demux1/2 -> Rate Transition6/1  "U2 CH3"
  Rate Transition5/1 -> Data Type Conversion/1  "U2 CH2"
  Demux2/1 -> Rate Transition4/1  "U2 CH2"
  Demux2/2 -> Rate Transition7/1  "U2 CH3"
  idq/1 -> Demux2/1
  vdq/1 -> Demux1/1

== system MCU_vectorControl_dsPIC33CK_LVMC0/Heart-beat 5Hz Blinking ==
  Delay : Delay  DelayLength=1  InitialCondition=0  SampleTime=.1
  Logical Operator : Logic  Operator=NOT  AllPortsSameDT=off  OutDataTypeStr=boolean
  Rate Transition2 : RateTransition  Deterministic=off  OutPortSampleTime=0.01
  LED1 : Outport  VectorParamsAs1DForOutWhenUnconnected=off
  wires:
  Rate Transition2/1 -> LED1/1
  Logical Operator/1 -> Rate Transition2/1, Delay/1
  Delay/1 -> Logical Operator/1

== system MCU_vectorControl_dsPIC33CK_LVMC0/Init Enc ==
  rho_cont : Inport
  Constant1 : Constant  Value=[0.5 0.5 0.5]  OutDataTypeStr=Inherit: Inherit via back propagation
  Constant2 : Constant  Value=[.6 .5 .5]  OutDataTypeStr=Inherit: Inherit via back propagation
  Data Type Duplicate : DataTypeDuplicate
  Rate Transition1 : RateTransition
  Rate Transition2 : RateTransition
  Rate Transition3 : RateTransition
  Switch : Switch  Criteria=u2 > Threshold
  Switch1 : Switch  Criteria=u2 > Threshold
  Wait 1s : Subsystem
  reset encoder : Outport
  PWM [0 1] : Outport  Port=2
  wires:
  Rate Transition2/1 -> Switch/2
  Rate Transition1/1 -> reset encoder/1
  Switch1/1 -> PWM [0 1]/1
  Constant1/1 -> Switch1/3
  Constant2/1 -> Switch/3
  Wait 1s/2(init done) -> Rate Transition2/1
  Switch/1 -> Data Type Duplicate/2, Switch1/1
  rho_cont/1 -> Switch/1, Data Type Duplicate/1
  Wait 1s/1(init enc) -> Rate Transition1/1
  [onoff] -> Wait 1s/Enable, Rate Transition3/1
  Rate Transition3/1 -> Switch1/2

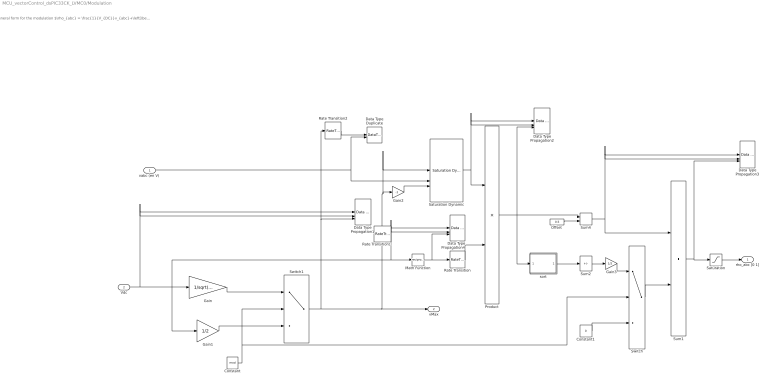
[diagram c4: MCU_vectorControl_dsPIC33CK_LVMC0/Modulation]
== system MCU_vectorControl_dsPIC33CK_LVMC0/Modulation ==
  note: General form for the modulation $\rho_{abc} = \frac{1}{V_{DC}}v_{abc}+\left[\begin{array}{c}1\\1\\1\end{array}\right]\lambda$ Sinusoidale modulation $\lambda = \frac{1}{2}$ it implies $V_{\rm max} = \frac{V_{\rm DC}}{2}$ Space Vector Modulation $\lambda = \frac{1}{2}\left(1-\frac{\min(v_{abc})+\max(v_{abc})}{V_{\rm DC}}\right)$ it implies $V_{\rm max} =\frac{V_{\rm DC}}{\sqrt{3}}$ For more details visits the ctrl+elec page dedicaded to the modulation
  "vabc (en V) " : Inport
  Vdc : Inport  Port=2
  Constant : Constant  Value=mod  OutDataTypeStr=boolean
  Constant1 : Constant  Value=0  OutDataTypeStr=Inherit: Inherit via back propagation
  Data Type Duplicate : DataTypeDuplicate
  Data Type Propagation1 : simulink/Signal Attributes/Data Type Propagation  PropDataType=fixdt(1, 16)  IfRefDouble=double  IfRefSingle=single  IsSigned=TRUE  NumBitsBase=max([NumBits1 NumBits2])  NumBitsMult=1  NumBitsAdd=0  NumBitsAllowFinal=[1:128]  PropScaling=2^-(15-ceil(log2(inverter.vDC/sqrt(3))))  ValuesUsedBestPrec=[100 -100]  SlopeBase=max([PosRange1 PosRange2])  SlopeMult=1/sqrt(3)  SlopeAdd=0  BiasBase=Bias1  BiasMult=1  BiasAdd=0
  Data Type Propagation2 : simulink/Signal Attributes/Data Type Propagation  PropDataType=fixdt(1, 16)  IfRefDouble=double  IfRefSingle=single  IsSigned=TRUE  NumBitsBase=max([NumBits1 NumBits2])  NumBitsMult=1  NumBitsAdd=0  NumBitsAllowFinal=[1:128]  PropScalingMode=Specify via dialog  PropScaling=2^-14  ValuesUsedBestPrec=[100 -100]  SlopeBase=Slope1/Slope2  SlopeMult=1  SlopeAdd=0  BiasBase=Bias1  BiasMult=1  BiasAdd=0
  Data Type Propagation3 : simulink/Signal Attributes/Data Type Propagation  PropDataType=fixdt(1, 16)  IfRefDouble=double  IfRefSingle=single  IsSigned=FALSE  NumBitsBase=max([NumBits1 NumBits2])  NumBitsMult=1  NumBitsAdd=0  NumBitsAllowFinal=[1:128]  PropScalingMode=Specify via dialog  PropScaling=2^-14  ValuesUsedBestPrec=[100 -100]  SlopeBase=Slope1/Slope2  SlopeMult=1  SlopeAdd=0  BiasBase=Bias1  BiasMult=1  BiasAdd=0
  Data Type Propagation4 : simulink/Signal Attributes/Data Type Propagation  PropDataType=fixdt(1, 16)  IfRefDouble=double  IfRefSingle=single  IsSigned=FALSE  NumBitsBase=max([NumBits1 NumBits2])  NumBitsMult=1  NumBitsAdd=0  NumBitsAllowFinal=[1:128]  PropScalingMode=Specify via dialog  PropScaling=2^-16  ValuesUsedBestPrec=[100 -100]  SlopeBase=max([PosRange1 PosRange2])  SlopeMult=1/sqrt(3)  SlopeAdd=0  BiasBase=Bias1  BiasMult=1  BiasAdd=0
  Gain : Gain  Gain=1/sqrt(3)
  Gain1 : Gain  Gain=1/2
  Gain2 : Gain  Gain=-1  ParamDataTypeStr=int16  OutDataTypeStr=Inherit: Inherit via back propagation
  Gain3 : Gain  Gain=1/2
  Math Function : Math  Operator=reciprocal  OutputSignalType=real  OutDataTypeStr=Inherit: Inherit via back propagation
  "Offset " : Constant  Value=0.5  OutMin=[0]  OutMax=[1]  OutDataTypeStr=Inherit: Inherit via back propagation
  Product : Product  Inputs=**  OutDataTypeStr=Inherit: Inherit via back propagation  SaturateOnIntegerOverflow=on
  Rate Transition : RateTransition
  Rate Transition1 : RateTransition
  Rate Transition2 : RateTransition
  Saturation : Saturate  UpperLimit=1  LowerLimit=0
  Saturation Dynamic : simulink/Discontinuities/Saturation Dynamic  OutMin=[]  OutMax=[]  OutDataTypeStr=Inherit: Same as second input  OutDataType=fixdt(1, 16)  OutScaling=2^-10  DoSatur=off
  Sum1 : Sum  OutMin=[0]  OutMax=[1]  OutDataTypeStr=Inherit: Inherit via back propagation  InputSameDT=on  SaturateOnIntegerOverflow=on
  Sum2 : Sum  Inputs=-  OutMin=[-1]  OutMax=[1]  InputSameDT=on  SaturateOnIntegerOverflow=on
  Sum4 : Sum  OutMin=[-1]  OutMax=[1]  InputSameDT=on  SaturateOnIntegerOverflow=on
  Switch : Switch  Criteria=u2 > Threshold
  Switch1 : Switch  Criteria=u2 > Threshold  OutDataTypeStr=Inherit: Inherit via back propagation
  sort : Subsystem
  rho_abc [0 1] : Outport  VectorParamsAs1DForOutWhenUnconnected=off
  vMax : Outport  Port=2  VectorParamsAs1DForOutWhenUnconnected=off
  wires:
  Rate Transition1/1 -> Gain2/1, Saturation Dynamic/1
  Rate Transition/1 -> Product/2
  "vabc (en V) "/1 -> Saturation Dynamic/2, Data Type Duplicate/2
  Constant/1 -> Switch/2, Switch1/2
  Switch1/1 -> Rate Transition2/1, Data Type Propagation1/3, vMax/1, Rate Transition1/1
  Math Function/1 -> Rate Transition/1, Data Type Propagation4/3
  Gain2/1 -> Saturation Dynamic/3
  Product/1 -> sort/1(In1), Sum4/1, Data Type Propagation2/3
  "Offset "/1 -> Sum4/2
  Switch/1 -> Sum1/2
  Constant1/1 -> Switch/3
  Sum4/1 -> Sum1/1, Data Type Propagation3/1, Data Type Propagation3/2
  Sum2/1 -> Gain3/1
  sort/1(MaxMin) -> Sum2/1
  Gain/1 -> Switch1/1
  Gain1/1 -> Switch1/3
  Saturation Dynamic/1 -> Data Type Propagation2/2, Data Type Propagation2/1, Product/1
  Saturation/1 -> rho_abc [0 1]/1
  Gain3/1 -> Switch/1
  Vdc/1 -> Gain1/1, Data Type Propagation4/1, Data Type Propagation4/2, Math Function/1, Gain/1, Data Type Propagation1/1, Data Type Propagation1/2
  Sum1/1 -> Data Type Propagation3/3, Saturation/1
  Rate Transition2/1 -> Data Type Duplicate/1

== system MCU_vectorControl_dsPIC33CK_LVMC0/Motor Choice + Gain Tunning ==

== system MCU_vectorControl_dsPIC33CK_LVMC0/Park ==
  xab(c) : Inport
  P(pth) : Inport  Port=2
  Clarke : Subsystem
  Park : Subsystem
  idq : Outport
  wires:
  P(pth)/1 -> Park/2(P(pth))
  Park/1(xdq) -> idq/1  "idq"
  xab(c)/1 -> Clarke/1(xab(c))
  Clarke/1(xalphabeta) -> Park/1(xalphabeta)

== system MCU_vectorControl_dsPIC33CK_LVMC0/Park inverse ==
  xdq : Inport
  P(pth) : Inport  Port=2
  Clarke Inverse : Subsystem
  Park inverse : Subsystem
  xabc : Outport
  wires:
  P(pth)/1 -> Park inverse/2(P(pth))
  Clarke Inverse/1(xabc) -> xabc/1
  xdq/1 -> Park inverse/1(xdq)
  Park inverse/1(xalpahbeta) -> Clarke Inverse/1(xalphabeta)

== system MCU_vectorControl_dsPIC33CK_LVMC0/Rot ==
  sin cos : Inport
  Demux3 : Demux  Outputs=2
  Gain : Gain  Gain=-1
  Mux1 : Mux
  Reshape : Reshape  OutputDimensionality=Customize  OutputDimensions=[2,2]
  "cos sin -sin cos " : Outport  PortDimensions=[2 2]
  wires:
  Demux3/2 -> Mux1/1, Mux1/4
  Demux3/1 -> Gain/1, Mux1/3
  Mux1/1 -> Reshape/1
  Gain/1 -> Mux1/2
  sin cos/1 -> Demux3/1
  Reshape/1 -> "cos sin -sin cos "/1
